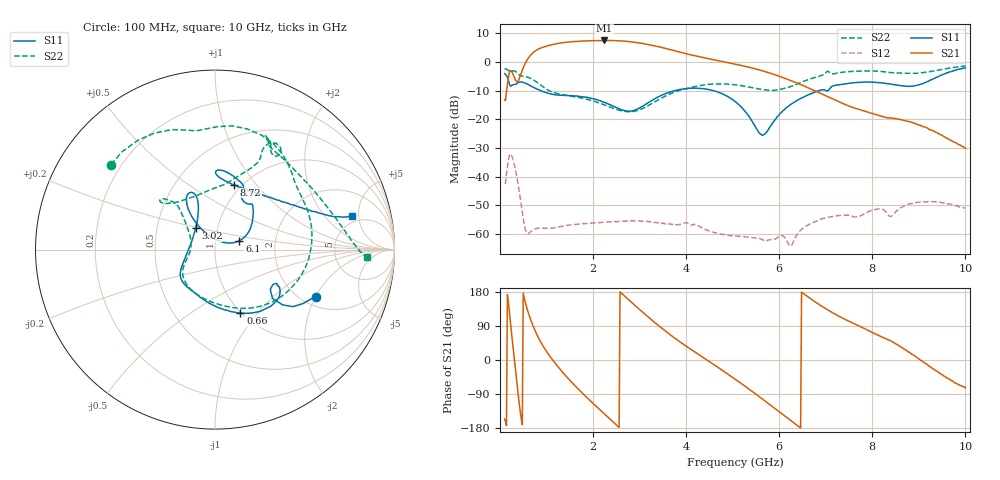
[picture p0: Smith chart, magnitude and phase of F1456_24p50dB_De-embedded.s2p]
! Integrated Device Technology
! Corporate Headquarters
! 6024 Silver Creek Valley Road
! San Jose, CA 95138  USA
! Phone:  1-408-284-8200
! Toll Free:  1-800-223-1366
! Webpage:  http://www.idt.com/
! Timing and RF Division
! 515 Groton Road, Suite 102
! Westford, MA 01886-6024
! Device:  F1456
! Description: 6-bit 0.5 dB Transmit Variable Gain Amplifier
! Frequency:  2100.0 -  2950.00 MHz
! Package:  6x6 mm Thin QFN Plastic Package: 28 pin
! State:  49
! Atten State:  24.5 dB
! Voltage:  +5.00 Volts
! Current:  216.946 mA
! Data:  The device was measured on a the F1455 evaluation board which has
!  individual transmission lines to the RF pins.  Data was collected
!  using a calibrated network analyzer.  The evaluation board was
!  de-embedded using a TRL calibration technique.
!  The reference plane is the edge of the package pin.
!  Pin  1 = CSb
!  Pin  2 = DATA
!  Pin  3 = CLK
!  Pin  4 = RSET
!  Pin  5 = GND
!  Pin  6 = RFIN  = Port 1
!  Pin  7 = GND
!  Pin  8 = NC
!  Pin  9 = NC
!  Pin 10 = NC
!  Pin 11 = NC
!  Pin 12 = NC
!  Pin 13 = NC
!  Pin 14 = /STBY
!  Pin 15 = GND
!  Pin 16 = RFOUT  = Port 2
!  Pin 17 = GND
!  Pin 18 = NC
!  Pin 19 = NC
!  Pin 20 = NC
!  Pin 21 = GND
!  Pin 22 = NC
!  Pin 23 = GND
!  Pin 24 = NC
!  Pin 25 = NC
!  Pin 26 = NC
!  Pin 27 = GND
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# GHz S dB R 50
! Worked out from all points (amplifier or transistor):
!   496 points, 100 MHz to 10 GHz, reference 50 ohm
!   highest |S21| = 7.4 dB at 2.24 GHz (marker M1)
!   |S21| within 3 dB of that: 825.8 MHz to 3.616 GHz (2.79 GHz wide, 126 % of centre)
!   unconditionally stable (mu >= 1): start of sweep to end of sweep
!   at 1.74 GHz: K = 128.21, MAG = 7.7 dB, |S12| = -56.4 dB
!   at 5.06 GHz: K = 478.68, MAG = 0.1 dB, |S12| = -60.6 dB
!   at 10 GHz: K = 625.30, MAG = -20.5 dB, |S12| = -51.0 dB
!   S11 on the Smith chart (normalised r, x): 100 MHz: 2.37, -2.02; 660 MHz: 0.99, -0.82; 3.02 GHz: 0.78, +0.19; 6.1 GHz: 1.31, +0.13; 8.72 GHz: 0.92, +0.78; 10 GHz: 4.18, +4.08
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0.1  -4.13 -24.9  -13.27 -156.1  -42.29 49.8  -2.52 140.8
0.24  -8.48 -31.0  -3.11 80.6  -32.25 -76.7  -3.43 94.5
0.32  -7.93 -29.6  -5.89 -8.1  -36.56 -154.6  -3.24 67.8
0.42  -7.03 -36.9  -5.61 -121.6  -45.72 140.7  -4.67 40.7
0.54  -7.40 -53.7  -0.66 154.7  -57.99 127.6  -5.12 16.6
0.66  -8.39 -68.2  2.33 106.4  -59.24 144.9  -5.78 -10.8
0.84  -9.81 -86.8  4.54 55.8  -57.87 117.0  -7.68 -48.5
1.16  -11.42 -113.3  6.11 -4.3  -57.84 80.2  -10.72 -94.4
1.48  -11.78 -130.5  6.90 -50.7  -56.89 58.2  -11.81 -123.3
1.76  -12.13 -140.6  7.20 -86.2  -56.38 43.4  -12.62 -139.3
2.24  -14.09 -156.1  7.43 -141.8  -55.88 23.2  -14.98 -157.6
2.62  -16.78 178.0  7.25 175.3  -55.53 8.0  -17.13 -175.6
3.02  -15.87 132.2  6.51 131.1  -55.56 -10.6  -16.53 156.5
3.4  -12.24 112.3  5.28 91.4  -56.00 -27.3  -13.29 138.2
4.12  -9.20 113.2  2.34 26.7  -56.97 -60.5  -8.87 131.8
5.06  -13.92 125.3  -0.83 -51.1  -60.64 -110.5  -8.04 138.7
5.64  -25.59 69.4  -3.15 -103.1  -61.98 -157.4  -9.69 123.2
6.1  -16.78 20.0  -5.65 -146.2  -60.85 163.8  -9.28 90.2
6.7  -10.99 41.5  -9.63 159.3  -56.14 148.3  -5.80 65.2
8.36  -7.69 88.2  -19.54 52.7  -53.71 66.9  -3.71 62.4
8.72  -8.46 73.6  -20.59 26.1  -49.91 69.4  -4.01 50.2
10  -2.11 13.8  -30.14 -73.6  -51.00 -23.4  -1.46 -2.6
